[IBIS Ver]   3.2
[File name]   sprm235b.ibs
[File Rev]   3.0
[Date]   Tuesday September 9, 2008
[Source]   File originated at Texas Instruments
[Notes]   Revision History:
   1.0: initial release, 12/21/07
   2.0: 2nd release, 07/31/08
   updated buffer models for
   BI2CSFZP18, BPCI33TPDFZP18
   BPCI33TPUFZP18, IQ33STCKP18PUSR50
   3.0: 3rd release, 09/09/2008
   updated buffer model from 3-state to I/O for
   BSSTL18WGFZ
   THIS IS RELEASE 3.0,THE CONTENTS ARE SUBJECT TO
   CHANGE WITHOUT PRIOR NOTICE,IF NECESSARY.
   Technology type SR50
   version : 3.3V version
   By default all models were done at 3.3V I/O supply besides
   some models associated with DDR interface have 1.8V tips
   Some pins have an input, output and a programmable pull
   associated with them.
   The [model selector] capability of IBIS ver 3.2 has been
   used on this ibis model.
   All the signal names do not contain nomenclature to indicate
   the active level
   For the pins, which are multiplexed with multiple functons,
   normally the reset default function or primary function is
   used for the pin name, for details on multiplexed functions,
   refer to Texas Instruments TMS320DM6437 Digital Media
   Processor data manual (TI literature number SPRS345).
   This file primarily contains the IBIS models for DDR interface
   and some other signals.
   This model passes IBIS syntax checker 4.1.0
   This model succeeds ICX parser syntax check
   IBIS syntax checker reports:
   Errors: 0
   Warnings: 144
   File Passed
   The warnings of "Pulldown Minimum/Typical/Maximum data is
   non-monotonic" are due to the dynamic output control circuit
   or feedback circuit of the buffers.
   The warnings of "Pullup Minimum/Typical/Maximum data is
   non-monotonic" are due to the ESD circuit, and/or damping
   resistor or dynamic output control circuit of the buffers.
   The warnings of "Model XXX: GND/POWER Clamp : Minimum/Typical
   /Maximum value never becomes zero" are caused by the clamp
   leakage.
   The warnings of "Model XXX: The [Falling Waveform]
   with [R_fixture]=XX Ohms and [V_fixture_xx]= XX V ..."
   are caused by either not sufficient simulation time
   for a waveform data or the waveform without the full
   rail-to-rail switching, the IBIS model accuracy has been
   validated against SPICE simulation.
[Disclaimer] Please be aware that in the absence of a written agreement
   Texas Instruments(TI) assumes no liability for:
   (1) The accuracy of the IBIS models provided to your company
   (2) The proper functioning of these Models in your design
   or for any resulting applications;or
   (3)Infringement of patents,copyrights or intellectual
   property rights resulting from your use of these models.
   TI provides IBIS Models as a service to our customers and
   therefore reserves the right to limit distribution of the
   Models.
[Copyright]   Property of Texas Instruments Incorporated.
   Unauthorised reproduction and/or distribution is strictly.
   prohibited.
   This product is protected under copyright law and trade
   secret law as an unpublished work.
   Created 2007,(C) Copyright 2007-2008,
   Texas Instruments Incorporated., All Rights Reserved.
   These commodities are under the U.S.
   Government distribution license control.As such,they are
   not to be re-exported without the prior approval of the
   U.S. Department of Commerce.
[Component]   c64lc_zdu_ddr
[Manufacturer]   Texas Instruments
[Package]
| variable   typ   min   max
R_pkg   3.74805e-001  2.32439e-001  5.33155e-001
L_pkg   5.68353e-009  4.00020e-009  7.74750e-009
C_pkg   1.53310e-012  1.20808e-012  2.00351e-012
[Pin]  signal_name   model_name   R_pin   L_pin   C_pin
W3   PCIEN   IT33SHYPDFZP18  3.50402e-001 5.27650e-009 1.45765e-012
V2   NTRST   IT33SHYPDFZP18  3.65959e-001 5.51440e-009 1.45027e-012
R2   PORZ   IT33SHYPUFZP18  3.91504e-001 5.67340e-009 1.55054e-012
T1   EMU0   BT3350CSHYPUFZP18 3.37284e-001 4.99560e-009 1.46359e-012
T3   RESETOUTN   OT3350BSFZP18   2.51388e-001 4.36960e-009 1.35671e-012
T2   EMU1   BT3350CSHYPUFZP18 3.12122e-001 4.79880e-009 1.40484e-012
R3   RESETN   IT33SHYPUFZP18  2.60273e-001 4.09300e-009 1.38316e-012
P2   I2C_DATA   BI2CSFZP18   2.96068e-001 4.68270e-009 1.33168e-012
P3   TINP1L   BT3350CSHYPUFZP18 2.56053e-001 4.11510e-009 1.33405e-012
N2   I2C_CLK   BI2CSFZP18   2.84961e-001 4.53630e-009 1.35940e-012
M3   GIO88   BT3350CSHYPUFZP18 2.32439e-001 4.00020e-009 1.24144e-012
R1   CLKOUT   BT3325ESHYPDFZSCP18  3.81360e-001 5.54960e-009 1.32193e-012
M2   GIO85   BT3350CSHYPUFZP18  2.86817e-001  4.37480e-009  1.36776e-012
N3   TOUT1L   BT3350CSHYPUFZP18  3.45359e-001  5.40410e-009  1.45040e-012
P1   GIO87   BT3350CSHYPUFZP18  3.88932e-001  5.67300e-009  1.39738e-012
N1   GIO86   BT3350CSHYPUFZP18  3.69384e-001  5.48490e-009  1.31395e-012
L2   TINP0L   BT3350CSHYPDFZP18  3.17172e-001  5.06890e-009  1.25940e-012
L3   TOUT0L   BT3350CSHYPDFZP18  2.87851e-001  4.49640e-009  1.32125e-012
K1   CLKR0   BT3350CSHYPDFZP18  3.55267e-001  5.19510e-009  1.27095e-012
K2   DX0   BT3350CSHYPDFZP18  3.21765e-001  4.84950e-009  1.39549e-012
J2   FSX0   BT3350CSHYPDFZP18  2.86890e-001  4.37710e-009  1.37322e-012
H2   FSR1   BT3350CSHYPDFZP18  2.88441e-001  5.12860e-009  1.37685e-012
K3   DR0   BT3350CSHYPDFZP18  2.37204e-001  4.05170e-009  1.29795e-012
J1   CLKX0   BT3350CSHYPDFZP18  3.81887e-001  5.84530e-009  1.33935e-012
H3   DR1   BT3350CSHYPDFZP18  2.91094e-001  4.47420e-009  1.30770e-012
H1   CLKR1   BT3350CSHYPDFZP18  3.64090e-001  5.41970e-009  1.27735e-012
J3   FSR0   BT3350CSHYPDFZP18  2.86957e-001  4.45830e-009  1.43030e-012
G2   DX1   BT3350CSHYPDFZP18  3.33099e-001  4.98300e-009  1.37685e-012
G1   CLKX1   BT3350CSHYPDFZP18  3.64218e-001  5.33300e-009  1.27190e-012
G3   FSX1   BT3350CSHYPDFZP18  3.56010e-001  5.24090e-009  1.49333e-012
F3   GIO4   BT3350CSHYPDFZP18  3.05672e-001  4.66100e-009  1.39048e-012
E1   GIO0   BPCI33TPDFZP18   4.56803e-001  6.56520e-009  1.63679e-012
D1   HCSN   BPCI33TPUFZP18   5.25162e-001  7.69700e-009  1.72339e-012
E2   GIO1   BPCI33TPDFZP18   4.20030e-001  6.22300e-009  1.71906e-012
D2   HINTN   BPCI33TPUFZP18   4.41426e-001  6.65940e-009  1.75880e-012
F1   GIO2   BPCI33TPDFZP18   4.77405e-001  7.24200e-009  1.77821e-012
C2   HDS2N   BPCI33TPUFZP18   4.48758e-001  6.62970e-009  1.81170e-012
F2   GIO3   BPCI33TPDFZP18   5.33155e-001  7.74750e-009  2.00351e-012
D3   HHWIL   BPCI33TPDFZP18   4.05764e-001  6.00830e-009  1.66715e-012
C1   HASN   BPCI33TPUFZP18   4.10285e-001  7.36130e-009  1.80970e-012
A5   HD11   BPCI33TPDFZP18   4.79897e-001  7.17980e-009  1.81759e-012
C3   HRDYN   BPCI33TPUFZP18   4.29782e-001  6.26320e-009  1.84705e-012
B2   HCNTLA   BPCI33TPDFZP18   4.52105e-001  6.57500e-009  1.90855e-012
C4   HCNTLB   BPCI33TPDFZP18   3.38587e-001  5.90900e-009  1.72006e-012
B3   HDS1N   BPCI33TPUFZP18   4.59394e-001  6.50650e-009  1.84956e-012
B5   HD14   BPCI33TPDFZP18   3.82226e-001  5.60880e-009  1.65807e-012
B4   HD13   BPCI33TPDFZP18   4.48908e-001  6.84590e-009  1.69649e-012
C5   HD12   BPCI33TPDFZP18   3.85721e-001  5.63540e-009  1.70731e-012
A3   HRW   BPCI33TPDFZP18   5.12319e-001  7.68450e-009  1.71812e-012
C7   HD06   BPCI33TPDFZP18   3.03915e-001  4.71690e-009  1.56121e-012
B6   HD10   BPCI33TPDFZP18   3.95205e-001  6.13000e-009  1.54250e-012
C9   HD01   BPCI33TPDFZP18   2.85939e-001  4.89150e-009  1.51737e-012
A4   HD15   BPCI33TPDFZP18   4.93929e-001  7.52330e-009  1.74769e-012
C6   HD09   BPCI33TPDFZP18   3.99895e-001  5.97250e-009  1.66259e-012
B7   HD07   BPCI33TPDFZP18   3.74444e-001  5.71130e-009  1.56265e-012
C8   HD04   BPCI33TPDFZP18   3.50069e-001  5.27970e-009  1.54502e-012
A6   HD08   BPCI33TPDFZP18   4.44430e-001  6.59320e-009  1.58117e-012
B10   EM_A_06   BPCI33TPDFZP18   2.98902e-001  5.24860e-009  1.48930e-012
A7   HD05   BPCI33TPDFZP18   4.61990e-001  6.98730e-009  1.58997e-012
B8   HD03   BPCI33TPDFZP18   3.76320e-001  5.64970e-009  1.55658e-012
A8   GIO57   BT3325ETHYPUFZSCP18  4.46964e-001 6.75620e-009 1.52637e-012
B9   HD00   BPCI33TPUFZP18   3.59476e-001  5.23060e-009  1.48070e-012
A10   EM_A_05   BPCI33TPDFZP18   3.98909e-001  5.96910e-009  1.38333e-012
A9   HD02   BPCI33TPDFZP18   4.01747e-001  6.38230e-009  1.52085e-012
C11   EM_A_09   BPCI33TPDFZP18   3.07717e-001  4.64010e-009  1.38231e-012
A11   EM_A_08   BPCI33TPDFZP18   3.95429e-001  6.01040e-009  1.33100e-012
C10   EM_A_07   BPCI33TPDFZP18   3.41101e-001  5.25420e-009  1.50019e-012
B11   EM_A_10   BPCI33TPDFZP18   3.57252e-001  5.39860e-009  1.41874e-012
C12   EM_A_11   BPCI33TPDFZP18   2.77770e-001  4.82950e-009  1.43285e-012
D12   AD26   BPCI33TPDFZP18   2.82752e-001  4.59420e-009  1.38084e-012
A12   CI7   BPCI33TPDFZP18   3.90384e-001  6.02220e-009  1.37379e-012
B12   EM_A_12   BPCI33TPDFZP18   3.33536e-001  5.04560e-009  1.35557e-012
A13   CI6   BPCI33TPDFZP18   3.85555e-001  5.63060e-009  1.28544e-012
B13   CI4   BPCI33TPDFZP18   3.37221e-001  5.12820e-009  1.41827e-012
C13   CI5   BPCI33TPDFZP18   3.20868e-001  4.85420e-009  1.39683e-012
A14   CI2   BPCI33TPDFZP18   3.79714e-001  5.66070e-009  1.36604e-012
B14   CI3   BPCI33TPDFZP18   3.60318e-001  5.48710e-009  1.42883e-012
D13   AD28   BPCI33TPDFZP18   2.68720e-001  4.16440e-009  1.52437e-012
C14   CI1   BPCI33TPDFZP18   3.15793e-001  4.87200e-009  1.37980e-012
D14   AD30   BPCI33TPDFZP18   2.92530e-001  4.96530e-009  1.43926e-012
C15   CI0   BPCI33TPDFZP18   3.26547e-001  4.99390e-009  1.42054e-012
C16   EM_A_21   BT3350CSHYPDFZP18  3.91971e-001  5.95520e-009  1.56826e-012
A15   YI7   BT3350CSHYPDFZP18  4.06317e-001  5.83820e-009  1.40085e-012
A17   VD   BT3350CSHYPDFZP18  3.62355e-001  5.16350e-009  1.47944e-012
B15   YI6   BT3350CSHYPDFZP18  4.69850e-001  6.87050e-009  1.61406e-012
B16   YI5   BT3350CSHYPDFZP18  4.21964e-001  6.07760e-009  1.63699e-012
A16   YI3   BT3350CSHYPDFZP18  4.55606e-001  6.75340e-009  1.60086e-012
A18   PCLK   BT3350CSHYPDFZP18  4.26060e-001  6.22340e-009  1.44085e-012
C17   C_WEN   BT3350CSHYPDFZP18  2.88652e-001  4.43680e-009  1.50156e-012
A19   HD   BT3350CSHYPDFZP18  4.49915e-001  6.71120e-009  1.50639e-012
B17   YI2   BT3350CSHYPDFZP18  4.23023e-001  6.20520e-009  1.72996e-012
B18   YI1   BT3350CSHYPDFZP18  4.45401e-001  6.54880e-009  1.69939e-012
C18   YI4   BT3350CSHYPDFZP18  3.72217e-001  5.31370e-009  1.66107e-012
C19   WRITE_WE   BT3350CSHYPUFZP18  3.98671e-001  5.76560e-009  1.71009e-012
B19   YI0   BT3350CSHYPDFZP18  4.57599e-001  6.57860e-009  1.78253e-012
A20   B1   BT3350CSHYPDFZP18  5.12647e-001  7.42070e-009  1.81534e-012
B20   G1   BT3350CSHYPDFZP18  4.10513e-001  5.91400e-009  1.67477e-012
B21   R0   BT3350CSHYPDFZP18  4.63465e-001  6.91680e-009  1.71848e-012
D19   READ_OE   BT3350CSHYPUFZP18  3.77061e-001  5.67610e-009  1.66261e-012
C21   R1   BT3350CSHYPDFZP18  4.17293e-001  6.09990e-009  1.51289e-012
C20   B2   BT3350CSHYPDFZP18  3.73396e-001  5.48200e-009  1.59887e-012
E21   COUT0   BT3350CSHYPDFZP18  3.68380e-001  5.56840e-009  1.50250e-012
E22   COUT2   BT3350CSHYPDFZP18  3.93883e-001  5.87240e-009  1.56092e-012
F20   COUT3   BT3350CSHYPDFZP18  3.29582e-001  4.96450e-009  1.52758e-012
D21   B0   BT3350CSHYPDFZP18  4.06366e-001  5.93970e-009  1.62823e-012
F21   COUT6   BT3350CSHYPDFZP18  3.02077e-001  5.04440e-009  1.38650e-012
D22   LCD_OE   BT3350CSHYPDFZP18  4.55417e-001  6.70600e-009  1.59839e-012
D20   WAIT_BSYN  BT3350CSHYPUFZP18  3.58416e-001  5.67010e-009  1.78574e-012
G20   COUT1   BT3350CSHYPDFZP18  3.21403e-001  5.09110e-009  1.55165e-012
E20   R2   BT3350CSHYPDFZP18  3.06058e-001  5.41580e-009  1.64628e-012
G21   COUT4   BT3350CSHYPDFZP18  3.49008e-001  5.32530e-009  1.49184e-012
J20   YOUT0_BOOTMODE0 BT3350CSHYPDFZP18 2.71641e-001 4.40800e-009 1.59269e-012
H21   YOUT3_BOOTMODE3 BT3350CSHYPDFZP18 2.76797e-001 4.88860e-009 1.26146e-012
C22   G0   BT3350CSHYPDFZP18  4.93245e-001  7.21960e-009  1.70280e-012
F22   COUT5   BT3350CSHYPDFZP18  4.10411e-001  5.97440e-009  1.41708e-012
G22   VCLK   BT3350DSHYPDFZSCP18 3.86289e-001 5.75430e-009  1.32809e-012
H20   COUT7   BT3350CSHYPDFZP18   2.92723e-001 5.33960e-009  1.41162e-012
K20   YOUT1_BOOTMODE1 BT3350CSHYPDFZP18 2.48778e-001 4.26140e-009 1.20808e-012
H22   VSYNC   BT3350CSHYPDFZP18   3.44659e-001 5.29700e-009  1.31708e-012
K19   YOUT4_FASTBOOT  BT3350CSHYPDFZP18 2.56887e-001 4.11250e-009 1.30367e-012
N22   MXI   IOSCHF18SHY   3.02656e-001  5.17920e-009  1.31672e-012
J21   YOUT6_8_16 BT3350CSHYPDFZP18  3.45206e-001  6.54250e-009  1.82153e-012
J22   HSYNC   BT3350CSHYPDFZP18  4.21085e-001  6.51330e-009  1.83332e-012
L20   YOUT2_BOOTMODE2 BT3350CSHYPDFZP18 3.00292e-001 5.34470e-009 1.48708e-012
K21   YOUT7   BT3350CSHYPDFZP18  4.40946e-001  6.92420e-009  1.84534e-012
K22   VPBECLK   BT3350CSHYPDFZP18  3.94679e-001  6.22790e-009  1.61206e-012
L19   YOUT5_LENDIAN   BT3350CSHYPUFZP18 2.84378e-001 4.46100e-009 1.43233e-012
Y22   DDR_D_31   BSSTL18WGFZ   4.41455e-001  6.44290e-009  1.61413e-012
AA21   DDR_D_30   BSSTL18WGFZ   4.66235e-001  6.90620e-009  1.71367e-012
Y21   DDR_D_29   BSSTL18WGFZ   4.30049e-001  6.22340e-009  1.71885e-012
AB20   DDR_D_28   BSSTL18WGFZ   4.45813e-001  6.43860e-009  1.62476e-012
Y18   DDR_DQM3   BSSTL18WGFZ   3.40998e-001  5.09730e-009  1.64235e-012
AA18   DDR_DQS3   BSSTL18WGFZ   3.65871e-001  5.50200e-009  1.64488e-012
Y20   DDR_D_27   BSSTL18WGFZ   4.49843e-001  6.68560e-009  1.66514e-012
AA20   DDR_D_26   BSSTL18WGFZ   4.80593e-001  6.80560e-009  1.64330e-012
AB19   DDR_D_25   BSSTL18WGFZ   4.46316e-001  6.61410e-009  1.47514e-012
Y19   DDR_D_24   BSSTL18WGFZ   4.31969e-001  6.24630e-009  1.65276e-012
AA19   DDR_D_23   BSSTL18WGFZ   4.60476e-001  6.50930e-009  1.52762e-012
AB18   DDR_D_22   BSSTL18WGFZ   4.19946e-001  6.05930e-009  1.37125e-012
AB17   DDR_D_21   BSSTL18WGFZ   3.87631e-001  5.84510e-009  1.47145e-012
Y17   DDR_D_20   BSSTL18WGFZ   3.17131e-001  4.96850e-009  1.48603e-012
AA15   DDR_DQS2   BSSTL18WGFZ   3.84967e-001  5.76510e-009  1.59344e-012
Y15   DDR_DQM2   BSSTL18WGFZ   3.04502e-001  4.88700e-009  1.57138e-012
AA17   DDR_D_19   BSSTL18WGFZ   3.92357e-001  5.86970e-009  1.59448e-012
AB16   DDR_D_18   BSSTL18WGFZ   4.19463e-001  6.06480e-009  1.47519e-012
Y16   DDR_D_17   BSSTL18WGFZ   3.34999e-001  5.11080e-009  1.52087e-012
AA16   DDR_D_16   BSSTL18WGFZ   3.72736e-001  5.48940e-009  1.44510e-012
AB15   DDR_A_00   BSSTL18WGFZ   4.01608e-001  6.08990e-009  1.35146e-012
AB14   DDR_A_01   BSSTL18WGFZ   4.04247e-001  5.89660e-009  1.42545e-012
Y14   DDR_A_02   BSSTL18WGFZ   3.98523e-001  5.80710e-009  1.59458e-012
AA14   DDR_A_03   BSSTL18WGFZ   4.29665e-001  6.28220e-009  1.53870e-012
AB13   DDR_A_04   BSSTL18WGFZ   3.66515e-001  5.72620e-009  1.50724e-012
Y13   DDR_A_05   BSSTL18WGFZ   3.18128e-001  4.87760e-009  1.44044e-012
AA13   DDR_A_06   BSSTL18WGFZ   4.21865e-001  6.05580e-009  1.51692e-012
AB12   DDR_A_07   BSSTL18WGFZ   4.05295e-001  6.09620e-009  1.42865e-012
Y12   DDR_A_08   BSSTL18WGFZ   3.18404e-001  4.78570e-009  1.46724e-012
AA12   DDR_A_09   BSSTL18WGFZ   3.21295e-001  4.96240e-009  1.41270e-012
AB11   DDR_A_10   BSSTL18WGFZ   3.89366e-001  6.17420e-009  1.37562e-012
AA11   DDR_A_11   BSSTL18WGFZ   3.56551e-001  5.25520e-009  1.44460e-012
AA10   DDR_A_12   BSSTL18WGFZ   3.18050e-001  4.76060e-009  1.50207e-012
AA9   DDR_BS_00   BSSTL18WGFZ   4.32347e-001  6.31100e-009  1.51686e-012
AB9   DDR_BS_01   BSSTL18WGFZ   4.08597e-001  5.92800e-009  1.38526e-012
AB10   DDR_BS_02   BSSTL18WGFZ   3.60853e-001  5.30380e-009  1.45455e-012
AB8   DDR_CLK0_N   BSSTL18WGFZ   4.05438e-001  5.87010e-009  1.39912e-012
AB7   DDR_CLK0   BSSTL18WGFZ   4.17756e-001  5.91050e-009  1.51107e-012
AA8   DDR_CKE   BSSTL18WGFZ   3.60517e-001  5.41390e-009  1.48672e-012
Y11   DDR_CS_N   BSSTL18WGFZ   3.57538e-001  5.40410e-009  1.60124e-012
Y10   DDR_WE_N   BSSTL18WGFZ   2.59498e-001  4.50290e-009  1.51635e-012
Y8   DDR_RAS_N   BSSTL18WGFZ   3.24292e-001  5.10980e-009  1.52379e-012
Y9   DDR_CAS_N   BSSTL18WGFZ   2.85176e-001  4.46200e-009  1.47460e-012
AB6   DDR_D_15   BSSTL18WGFZ   4.22753e-001  6.23830e-009  1.43842e-012
Y6   DDR_D_14   BSSTL18WGFZ   3.67723e-001  5.60450e-009  1.61981e-012
AA6   DDR_D_13   BSSTL18WGFZ   3.85076e-001  5.79290e-009  1.56360e-012
AB5   DDR_D_12   BSSTL18WGFZ   4.09269e-001  6.17890e-009  1.59596e-012
Y7   DDR_DQM1   BSSTL18WGFZ   2.69162e-001  4.76200e-009  1.43847e-012
AA7   DDR_DQS1   BSSTL18WGFZ   3.46563e-001  5.29750e-009  1.60426e-012
Y5   DDR_D_11   BSSTL18WGFZ   3.68694e-001  5.50250e-009  1.64866e-012
AA5   DDR_D_10   BSSTL18WGFZ   4.16485e-001  6.22080e-009  1.59128e-012
W5   DDR_D_09   BSSTL18WGFZ   3.40409e-001  5.13000e-009  1.73494e-012
AB4   DDR_D_08   BSSTL18WGFZ   4.46437e-001  6.44490e-009  1.49494e-012
W4   DDR_D_07   BSSTL18WGFZ   3.99431e-001  6.04990e-009  1.67614e-012
AB3   DDR_D_06   BSSTL18WGFZ   4.65557e-001  6.73050e-009  1.55413e-012
Y3   DDR_D_05   BSSTL18WGFZ   4.95306e-001  7.01100e-009  1.95743e-012
AA3   DDR_D_04   BSSTL18WGFZ   4.29556e-001  6.12400e-009  1.90869e-012
AA4   DDR_DQS0   BSSTL18WGFZ   3.86310e-001  5.75510e-009  1.85437e-012
Y4   DDR_DQM0   BSSTL18WGFZ   3.22816e-001  5.49850e-009  1.74192e-012
AA2   DDR_D_03   BSSTL18WGFZ   4.96975e-001  7.00370e-009  1.72454e-012
W2   DDR_D_02   BSSTL18WGFZ   3.88729e-001  5.64340e-009  1.66019e-012
Y2   DDR_D_01   BSSTL18WGFZ   4.16496e-001  6.12420e-009  1.63261e-012
Y1   DDR_D_00   BSSTL18WGFZ   4.46604e-001  6.56140e-009  1.53478e-012
U3   TDI   IT33SHYPUFZP18   3.30353e-001  4.96520e-009  1.43344e-012
U1   TCK   IQ33STCKP18PUSR50 3.39696e-001 5.83100e-009  1.49000e-012
V3   TMS   IT33SHYPUFZP18   3.99748e-001 5.61610e-009  1.60300e-012
U2   TDO   OT3350CSFZP18   3.20929e-001  4.94540e-009 1.40757e-012
[Model Selector]   IT33SHYPDFZP18
IT33SHYPDFZP18_PD   Cell operated with Pulldown"on"
IT33SHYPDFZP18_Z   Cell operated with Pulldown "off"
[Model Selector]   IT33SHYPUFZP18
IT33SHYPUFZP18_PU   Cell operated with Pullup "on"
IT33SHYPUFZP18_Z   Cell operated with Pullup "off"
[Model Selector]   BT3350CSHYPUFZP18
BT3350CSHYPUFZP18_PU   Cell operated with Pullup "on"
BT3350CSHYPUFZP18_Z   Cell operated with Pullup "off"
[Model Selector]   BT3325ESHYPDFZSCP18
BT3325ESHYPD_PD  Cell operated with Pulldown"on"
BT3325ESHYPD_Z   Cell operated with Pulldown "off"
[Model Selector]   BT3350CSHYPDFZP18
BT3350CSHYPDFZP18_PD   Cell operated with Pulldown"on"
BT3350CSHYPDFZP18_Z   Cell operated with Pulldown "off"
[Model Selector]   BPCI33TPDFZP18
BPCI33TPDFZP18_PD   Cell operated with Pulldown"on"
BPCI33TPDFZP18_Z   Cell operated with Pulldown"off"
[Model Selector]   BPCI33TPUFZP18
BPCI33TPUFZP18_PU   Cell operated with Pullup"on"
BPCI33TPUFZP18_Z   Cell operated with Pullup"off"
[Model Selector]   BT3325ETHYPUFZSCP18
BT3325ETHYPU_PU  Cell operated with Pullup"on"
BT3325ETHYPU_Z   Cell operated with Pullup"off"
[Model Selector]   BT3350DSHYPDFZSCP18
BT3350DSHYPD_PD  Cell operated with Pulldown"on"
BT3350DSHYPD_Z   Cell operated with Pulldown "off"
[Model Selector]   IQ33STCKP18PUSR50
IQ33STCKP18PUSR50_PU   Cell operated with Pullup"on"
IQ33STCKP18PUSR50_Z   Cell operated with Pullup"off"
| Models and submodels in the file (25): OT3350CSFZP18 (3-state), IQ33STCKP18PUSR50_PU (Input), IQ33STCKP18PUSR50_Z (Input), BSSTL18WGFZ (I/O), IOSCHF18SHY (Input), BT3350DSHYPD_Z (I/O), BT3350DSHYPD_PD (I/O), BT3325ETHYPU_Z (I/O), BT3325ETHYPU_PU (I/O), BPCI33TPUFZP18_PU (I/O), BPCI33TPUFZP18_Z (I/O), BPCI33TPDFZP18_PD (I/O), BPCI33TPDFZP18_Z (I/O), BT3350CSHYPDFZP18_PD (I/O), BT3350CSHYPDFZP18_Z (I/O), BT3325ESHYPD_Z (I/O), BT3325ESHYPD_PD (I/O), BI2CSFZP18 (I/O_open_drain), OT3350BSFZP18 (3-state), BT3350CSHYPUFZP18_PU (I/O), BT3350CSHYPUFZP18_Z (I/O), IT33SHYPUFZP18_PU (Input), IT33SHYPUFZP18_Z (Input), IT33SHYPDFZP18_PD (Input), IT33SHYPDFZP18_Z (Input)
